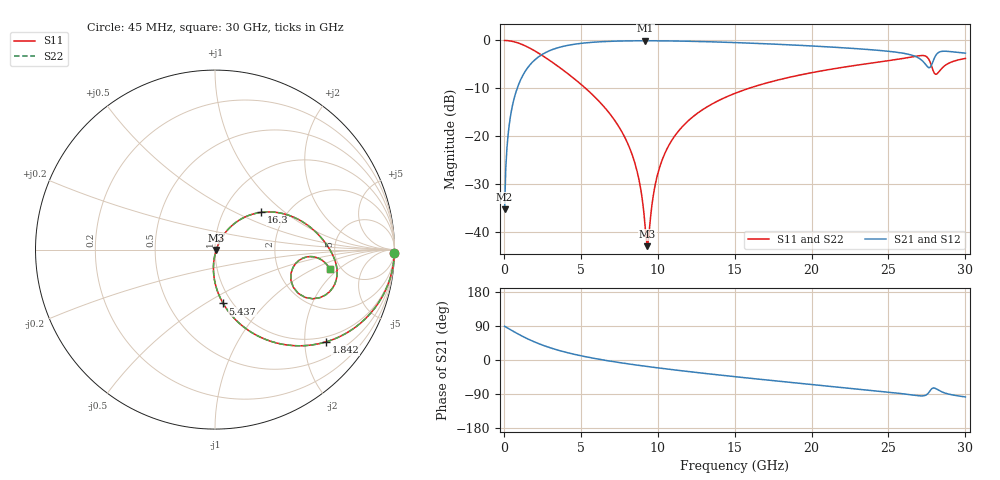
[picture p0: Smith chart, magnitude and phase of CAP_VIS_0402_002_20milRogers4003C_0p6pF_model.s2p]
! S-parameter model data by Modelithics Inc.  support@modelithics.com  813-866-6335  Tampa FL USA
! S-Parameter data specifications:
! Substrate: 20-mil Rogers 4003C, substrate thickness, H=0.508mm, Dielectric constant, Er=3.75
! PCB Mounting Pad Footprint: Pad width, PadW=0.50mm , Pad length, PadL=0.50mm , Pad gap, PadG (edge-to-edge)=0.40mm , Reference planes=1.4mm apart
! Created Wed Nov 18 12:40:32 2015
# hz S ma R 50
! 2 Port Network Data from SP1.SP block
! freq  magS11  angS11  magS21  angS21  magS12  angS12  magS22  angS22
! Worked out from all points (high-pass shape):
!   401 points, 45 MHz to 30 GHz, reference 50 ohm
!   highest |S21| = -0.06 dB at 9.181 GHz (marker M1); lowest = -35.3 dB at 45 MHz (marker M2)
!   |S21| within 3 dB of the highest: 2.418 GHz to 26.51 GHz (24.09 GHz wide, 167 % of centre); 28.09 GHz to end of sweep
!   lowest |S11| = -43.0 dB at 9.331 GHz (marker M3), VSWR 1.01, Z = 50.7 - j0.2 ohm
!   |S11| at or under -10 dB: 5.31 GHz to 15.92 GHz (10.61 GHz wide, 100 % of centre)
!   |S22| runs from -43.0 to 0.0 dB; largest |S21 - S12| = 0
!   S11 on the Smith chart (normalised r, x): 45 MHz: open; 1.842 GHz: 0.86, -2.52; 5.437 GHz: 0.91, -0.60; 16.3 GHz: 1.50, +0.70; 30 GHz: 4.10, -1.52
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4.5e7  0.9998 -1.1  0.01725 88.9  0.01725 88.9  0.9998 -1.1
2.696625e8  0.9947 -6.4  0.1029 83.6  0.1029 83.6  0.9947 -6.4
5.692125e8  0.9767 -13.4  0.2139 76.6  0.2139 76.6  0.9767 -13.4
1.8423e9  0.8052 -39.6  0.591 50.2  0.591 50.2  0.8052 -39.6
3.34005e9  0.5626 -61.6  0.8232 28.1  0.8232 28.1  0.5626 -61.6
5.062462e9  0.3426 -78.5  0.9345 10.7  0.9345 10.7  0.3426 -78.5
5.4369e9  0.3031 -81.4  0.9477 7.6  0.9477 7.6  0.3031 -81.4
8.13285e9  0.07804 -95.7  0.9902 -10.5  0.9902 -10.5  0.07804 -95.7
8.73195e9  0.03819 -93.6  0.9922 -14.0  0.9922 -14.0  0.03819 -93.6
9.181275e9  0.01149 -68.6  0.9926 -16.4  0.9926 -16.4  0.01149 -68.6
9.33105e9  0.007107 -16.1  0.9926 -17.2  0.9926 -17.2  0.007107 -16.1
1.007992e10  0.04491 59.4  0.9913 -21.1  0.9913 -21.1  0.04491 59.4
1.172745e10  0.1323 57.3  0.9828 -29.2  0.9828 -29.2  0.1323 57.3
1.50225e10  0.2804 44.1  0.9502 -44.1  0.9502 -44.1  0.2804 44.1
1.629559e10  0.3306 38.9  0.9337 -49.5  0.9337 -49.5  0.3306 38.9
2.003996e10  0.4618 23.9  0.8754 -64.7  0.8754 -64.7  0.4618 23.9
2.505742e10  0.6173 3.3  0.7688 -85.1  0.7688 -85.1  0.6173 3.3
2.707939e10  0.6945 -11.8  0.637 -94.6  0.637 -94.6  0.6945 -11.8
2.76036e10  0.6423 -24.7  0.521 -86.7  0.521 -86.7  0.6423 -24.7
2.797804e10  0.4557 -21.9  0.6517 -73.9  0.6517 -73.9  0.4557 -21.9
2.842736e10  0.5035 -4.9  0.7675 -83.4  0.7675 -83.4  0.5035 -4.9
3e10  0.6488 -9.5  0.7367 -97.5  0.7367 -97.5  0.6488 -9.5
